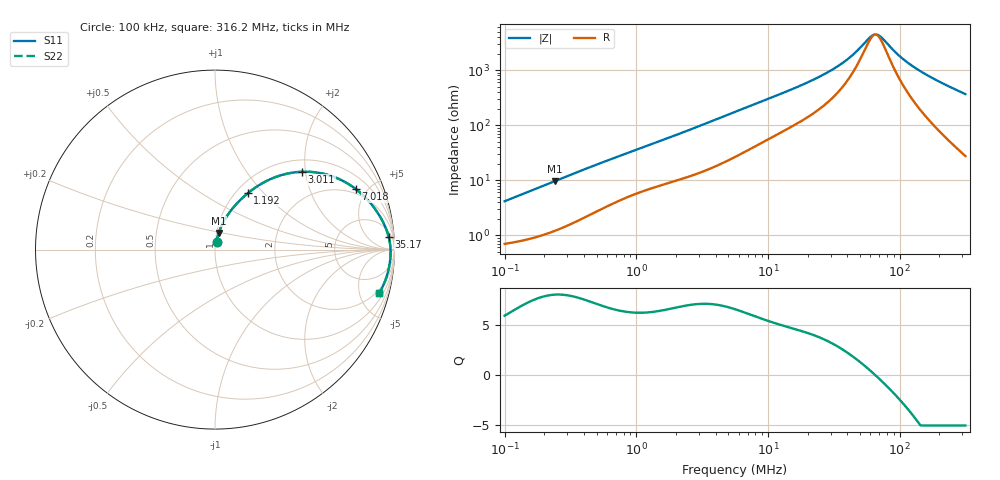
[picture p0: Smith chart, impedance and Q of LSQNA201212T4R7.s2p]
! LSQNA201212T4R7  S-PARAMETER MODEL  ( General Type )
! Model Generated by TAIYO YUDEN Corporation (http://www.ty-top.com)
! Version 2.0
! TAIYO YUDEN Control No. 100810NF25SB-FKC
! Copyright(c) 2007 TAIYO YUDEN CO.,LTD. All Rights Reserved.
! Product Description (link to TY-COMPAS)
! https://ds.yuden.co.jp/TYCOMPAS/or/detail?pn=LSQNA201212T4R7M&u=M
! Products Name : Inductors
! Characteristics :
!  Inductance : 4.7 uH , SRF(min) : 45 MHz , DC Resistance(max) : 0.52 Ohm
!  Rated Current : Saturation :300 mA , Temp Rise : 580 mA (40 degC)
!  Case Size : 2.0 x 1.25 / 0.079 x 0.049 [mm/inch] , Thickness : 1.25 / 0.049 [mm/inch]
!  (Conditions: Temperature = 25 degC , DC Bias Current/Voltage = 0A / 0V)
! External Node Assignments :
!  1  o---GGG---o  2
! GND o---------o GND
! Frequency Range : 0.1MHz  -  316.199832MHz  [ 402 STEP ]
# MHz S RI R 50
! Freq[MHz].  S11 Real  S11 Imag  S21 Real  S21 Imag  S12 Real  S12 Imag  S22 Real  S22 Imag
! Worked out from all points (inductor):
!   401 points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, 100 kHz to 316.2 MHz, reference 50 ohm
!   read as one part in series: L = 6.45 uH near 104.1 kHz
!   highest Q = 7.97 at 242.7 kHz (marker M1), where L = 6.33 uH
!   self-resonance near 65.32 MHz
!   S11 on the Smith chart (normalised r, x): 100 kHz: 1.01, +0.08; 1.192 MHz: 1.13, +0.82; 3.011 MHz: 1.27, +1.91; 7.018 MHz: 1.70, +4.24; 35.17 MHz: 10, +23; 316.2 MHz: 1.55, -7.32
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0.1  0.00855 0.0403  0.9915 -0.0403  0.9915 -0.0403  0.00855 0.0403
0.242659  0.0209 0.0933  0.9791 -0.0933  0.9791 -0.0933  0.0209 0.0933
0.385695  0.0402 0.141  0.9598 -0.141  0.9598 -0.141  0.0402 0.141
0.705896  0.0949 0.2256  0.9051 -0.2256  0.9051 -0.2256  0.0949 0.2256
1.191896  0.183 0.3143  0.817 -0.3143  0.817 -0.3143  0.183 0.3143
1.487603  0.2364 0.3533  0.7636 -0.3533  0.7636 -0.3533  0.2364 0.3533
3.01116  0.4842 0.4338  0.5158 -0.4338  0.5158 -0.4338  0.4842 0.4338
4.073637  0.6075 0.4218  0.3925 -0.4218  0.3925 -0.4218  0.6075 0.4218
5.623165  0.723 0.3774  0.277 -0.3774  0.277 -0.3774  0.723 0.3774
7.018265  0.7863 0.3359  0.2137 -0.3359  0.2137 -0.3359  0.7863 0.3359
11.61388  0.8832 0.2377  0.1168 -0.2377  0.1168 -0.2377  0.8832 0.2377
21.68824  0.945 0.1352  0.055 -0.1352  0.055 -0.1352  0.945 0.1352
35.17403  0.9677 0.0709  0.0323 -0.0709  0.0323 -0.0709  0.9677 0.0709
43.90066  0.9733 0.0446  0.0267 -0.0446  0.0267 -0.0446  0.9733 0.0446
58.20626  0.9772 0.0128  0.0228 -0.0128  0.0228 -0.0128  0.9772 0.0128
63.09128  0.9778 0.00386  0.0222 -0.00386  0.0222 -0.00386  0.9778 0.00386
69.77805  0.9782 -0.00737  0.0218 0.00737  0.0218 0.00737  0.9782 -0.00737
83.65039  0.9781 -0.0279  0.0219 0.0279  0.0219 0.0279  0.9781 -0.0279
104.4039  0.9764 -0.0544  0.0236 0.0544  0.0236 0.0544  0.9764 -0.0544
138.4253  0.9711 -0.0918  0.0289 0.0918  0.0289 0.0918  0.9711 -0.0918
202.9849  0.9556 -0.1529  0.0444 0.1529  0.0444 0.1529  0.9556 -0.1529
316.1998  0.9151 -0.2438  0.0849 0.2438  0.0849 0.2438  0.9151 -0.2438
